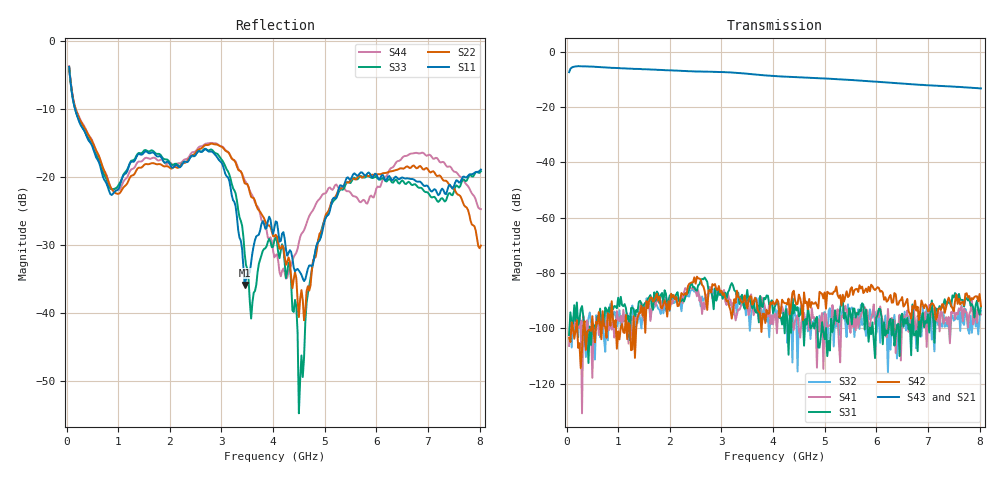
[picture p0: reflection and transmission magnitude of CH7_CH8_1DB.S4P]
!Agilent Technologies,E5071C,MY46316741,A.11.02
!Date: Mon Jun 01 10:30:03 2026
!Data & Calibration Information:
!1:CH7 INPUT 2:CH7 OUTPUT 3:CH8 INPUT 4:CH8 OUTPUT
!Freq	S11:SOLT4(ON)	S12:SOLT4(ON)	S13:SOLT4(ON)	S14:SOLT4(ON)
!	S21:SOLT4(ON)	S22:SOLT4(ON)	S23:SOLT4(ON)	S24:SOLT4(ON)
!	S31:SOLT4(ON)	S32:SOLT4(ON)	S33:SOLT4(ON)	S34:SOLT4(ON)
!	S41:SOLT4(ON)	S42:SOLT4(ON)	S43:SOLT4(ON)	S44:SOLT4(ON)
!PortZ  Port1:50+j0  Port2:50+j0  Port3:50+j0  Port4:50+j0
!Above PortZ is port z conversion or system Z0 setting when saving the data.
!When reading, reference impedance value at option line is always used.
# Hz S dB R 50
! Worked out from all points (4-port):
!   320 points, 50 MHz to 8.025 GHz, reference 50 ohm
!   strongest paths, dB at 50 MHz, 2.05 GHz, 4.05 GHz, 6.05 GHz, 8.025 GHz:
!     S43: -7.3, -6.7, -8.8, -10.9, -13.2
!     S21: -7.4, -6.8, -8.9, -11.1, -13.4
!     S42: -103.5, -88.6, -90.9, -85.4, -92.0
!     S31: -102.4, -87.9, -91.5, -92.9, -92.1
!     S41: -106.3, -91.0, -94.8, -95.9, -94.9
!     S32: -102.3, -88.5, -93.2, -95.5, -93.7
!   lowest |S11| = -35.9 dB at 3.45 GHz (marker M1), VSWR 1.03, Z = 49.1 - j1.33 ohm
!   |S11| at or under -10 dB: 165.6 MHz to end of sweep
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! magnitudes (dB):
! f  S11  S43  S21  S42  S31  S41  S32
! 50 MHz  -3.8  -7.3  -7.4  -103.5  -102.4  -106.3  -102.3
! 875 MHz  -22.6  -5.8  -5.8  -90.2  -93.5  -100.4  -95.5
! 3.45 GHz  -35.9  -7.8  -8.0  -88.1  -92.9  -88.2  -90.1
! 4.325 GHz  -30.7  -9.0  -9.2  -94.8  -94.3  -95.4  -96.5
! 4.5 GHz  -33.8  -9.2  -9.3  -87.8  -95.6  -100.4  -94.5
! 5.3 GHz  -21.2  -9.9  -10.1  -87.9  -92.7  -112.2  -98.3
! 8.025 GHz  -18.9  -13.2  -13.4  -92.0  -92.1  -94.9  -93.7
